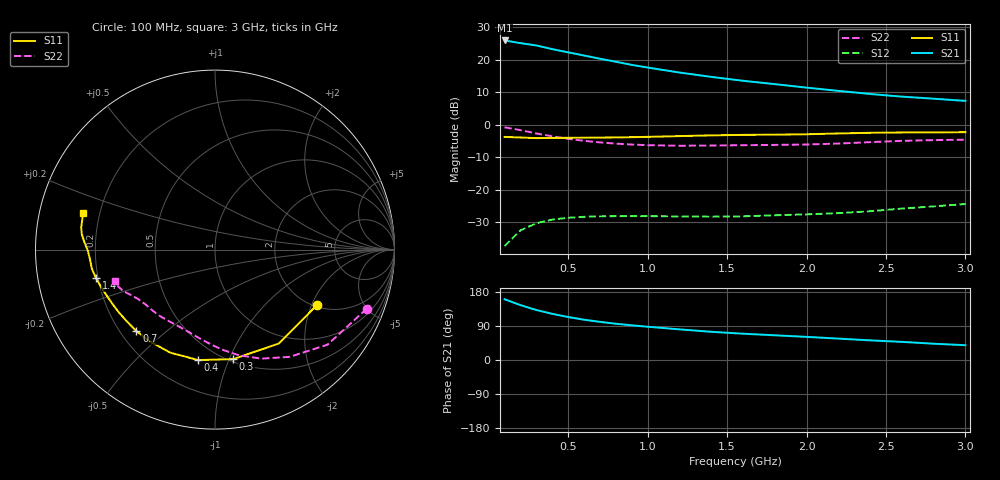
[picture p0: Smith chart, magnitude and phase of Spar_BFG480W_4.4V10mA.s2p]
! Filename: 4_410BFG480.001
! Title: BFG480W
! Bias: Vce=4.4V; Ic=10mA
! Company: NXP Semiconductors NL
! User: Quality&Reliability T&D
! Measure time: 10 Nov 1999 / 12:05:15
#  MHz  S  MA  R 50
! Freq  S11  S21  S12  S22  :
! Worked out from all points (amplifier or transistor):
!   20 points, 100 MHz to 3 GHz, reference 50 ohm
!   highest |S21| = 25.9 dB at 100 MHz (marker M1)
!   |S21| within 3 dB of that: start of sweep to 433.4 MHz
!   unconditionally stable (mu >= 1): 1.668 GHz to end of sweep
!   at 400 MHz: K = 0.25, MSG = 26.2 dB, |S12| = -29.2 dB
!   at 1.2 GHz: K = 0.74, MSG = 22.1 dB, |S12| = -28.3 dB
!   at 3 GHz: K = 1.14, MAG = 13.6 dB, |S12| = -24.5 dB
!   S11 on the Smith chart (normalised r, x): 100 MHz: 2.04, -2.18; 300 MHz: 0.52, -1.04; 400 MHz: 0.39, -0.78; 700 MHz: 0.26, -0.40; 1.4 GHz: 0.19, -0.11; 3 GHz: 0.14, +0.13
100  0.6457 -28.8  19.71 160.3  0.01344 65.3  0.9076 -21.2
200  0.6327 -55.8  17.92 144.8  0.02357 55.1  0.8206 -40.2
300  0.6185 -80.5  16.5 131.8  0.03031 46.6  0.729 -55.0
400  0.6226 -98.6  14.5 121.8  0.03452 39.9  0.6598 -67.0
500  0.626 -113.5  12.92 113.4  0.03672 35.3  0.6039 -77.2
600  0.627 -125.2  11.56 106.3  0.03808 32.2  0.5621 -85.1
700  0.6308 -134.0  10.31 100.7  0.0387 30.3  0.5316 -91.8
800  0.6338 -141.3  9.269 95.7  0.0389 29.3  0.5088 -97.6
900  0.6396 -146.8  8.292 91.5  0.03891 29.0  0.4929 -102.9
1000  0.6467 -152.1  7.547 87.8  0.03893 29.2  0.4816 -107.9
1200  0.6644 -160.4  6.324 80.8  0.03858 30.8  0.4725 -116.8
1400  0.6819 -166.5  5.42 74.4  0.03818 33.6  0.4754 -124.2
1600  0.6942 -171.1  4.721 69.4  0.03868 38.3  0.4813 -130.0
1800  0.6988 -175.6  4.191 65.2  0.04012 43.5  0.4862 -135.6
2000  0.709 -179.6  3.703 61.0  0.04147 48.5  0.493 -141.6
2200  0.7298 176.6  3.304 56.4  0.04335 53.1  0.5103 -147.5
2400  0.747 173.4  2.958 51.8  0.04636 56.9  0.5365 -152.3
2600  0.7556 170.7  2.691 47.8  0.05092 60.3  0.5616 -155.7
2800  0.7575 167.8  2.502 43.0  0.05502 62.0  0.576 -158.9
3000  0.7639 164.5  2.315 39.0  0.0599 64.0  0.5857 -162.8
